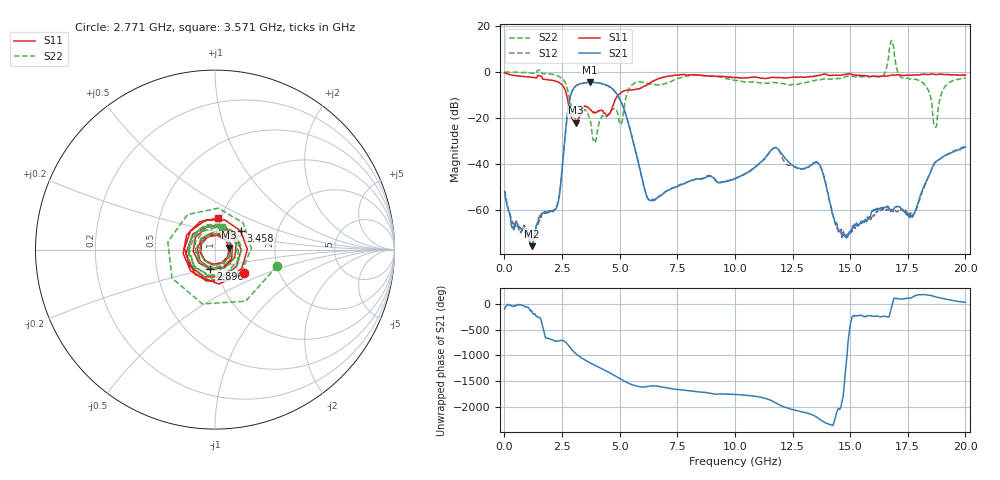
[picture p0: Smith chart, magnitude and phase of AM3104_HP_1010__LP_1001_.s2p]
!Created with skrf (http://scikit-rf.org).
# Hz S RI R 50.0
!freq ReS11 ImS11 ReS21 ImS21 ReS12 ImS12 ReS22 ImS22
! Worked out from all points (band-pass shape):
!   1601 points, 10 MHz to 20 GHz, reference 50 ohm
!   highest |S21| = -4.48 dB at 3.708 GHz (marker M1); lowest = -75.7 dB at 1.184 GHz (marker M2)
!   |S21| within 3 dB of the highest: 2.979 GHz to 4.706 GHz (1.727 GHz wide, 44.9 % of centre)
!   lowest |S11| = -22.0 dB at 3.096 GHz (marker M3), VSWR 1.17, Z = 58.5 + j1.21 ohm
!   |S11| at or under -10 dB: 2.7 GHz to 4.948 GHz (2.247 GHz wide, 58.8 % of centre)
!   |S22| runs from -30.8 to 13.7 dB; largest |S21 - S12| = 0.048
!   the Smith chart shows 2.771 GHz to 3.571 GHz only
!   S11 on the Smith chart (normalised r, x): 2.771 GHz: 1.33, -0.36; 2.896 GHz: 0.93, -0.20; 3.458 GHz: 1.30, +0.28; 3.571 GHz: 0.97, +0.35
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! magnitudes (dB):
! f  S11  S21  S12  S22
! 10 MHz  -0.4  -52.1  -51.5  0.0
! 1.184 GHz  -2.3  -75.7  -72.5  -0.6
! 2.296 GHz  -4.2  -58.0  -57.5  -1.7
! 2.771 GHz  -13.6  -15.7  -15.7  -8.9
! 2.896 GHz  -19.2  -9.5  -9.5  -14.9
! 3.096 GHz  -22.0  -6.1  -6.1  -21.1
! 3.346 GHz  -16.7  -5.0  -5.1  -17.4
! 3.458 GHz  -15.0  -4.8  -4.8  -16.6
! 3.571 GHz  -15.1  -4.6  -4.7  -17.7
! 3.708 GHz  -16.1  -4.5  -4.6  -21.0
! 4.92 GHz  -10.3  -10.3  -10.3  -18.5
! 6.169 GHz  -5.8  -53.7  -53.8  -4.9
! 6.682 GHz  -3.0  -54.3  -54.5  -5.6
! 10.01 GHz  -2.5  -46.6  -46.5  -3.7
! 11.72 GHz  -2.4  -32.9  -33.0  -4.6
! 13.34 GHz  -2.1  -40.2  -40.2  -4.0
! 14.74 GHz  -1.2  -70.9  -70.9  -2.3
! 16.68 GHz  -1.6  -59.0  -59.7  7.3
! 17.7 GHz  -1.5  -63.0  -62.2  -3.2
! 18.69 GHz  -1.1  -39.2  -39.3  -23.8
! 19.11 GHz  -1.1  -36.2  -36.4  -6.4
! 20 GHz  -1.3  -32.7  -32.2  -2.6
